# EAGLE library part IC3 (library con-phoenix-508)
PHOENIX
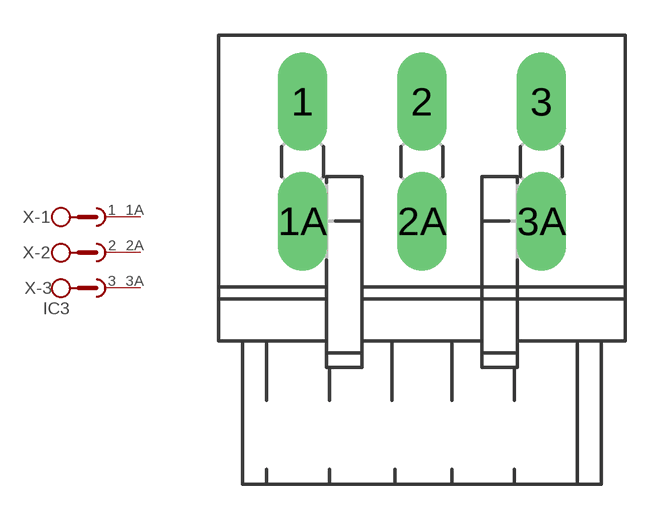
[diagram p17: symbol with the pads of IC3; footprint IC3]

Designator prefix X; gates -1=SKB2 -2=SKB2 -3=SKB2V

## IC3 (OC_FARNELL: unknown; OC_NEWARK: unknown)  [IC3]
1  -1:1  pas
1A  -1:2  pas
2  -2:1  pas
2A  -2:2  pas
3  -3:1  pas
3A  -3:2  pas

## Footprint IC3 (pad centres in mm)
PHOENIX
drill 1.397 long: 1 -5.08,2.54; 1A -5.08,-2.54; 2 0,2.54; 2A 0,-2.54; 3 5.08,2.54; 3A 5.08,-2.54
